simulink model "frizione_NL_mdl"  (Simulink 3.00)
settings: Solver=ode23s  StartTime=0.0  StopTime=10.0  RelTol=1e-10
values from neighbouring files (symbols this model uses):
  A = 4*(cm^2)    (= 0.0004)    [frizione_NL.m]
  b = 0.25*10^2*N*sec/m    (= 25)    [frizione_NL.m]
  Cm = 1*(cm^3)/(50*bar)    (= 2e-13)    [frizione_NL.m]
  Ic = Ic_max    (= 0.01)    [frizione_NL.m]
  K_x = [0:0.01:1]*3*mm    [frizione_NL.m]
  K_y = polyval(P,K_x)    [frizione_NL.m]
  mp = 0.3*Kg    (= 0.3)    [frizione_NL.m]
  P10 = 0*bar    (= 0)    [frizione_NL.m]
  Pm = 50*bar    (= 5000000)    [frizione_NL.m]
  x0 = 0*cm    (= 0)    [frizione_NL.m]

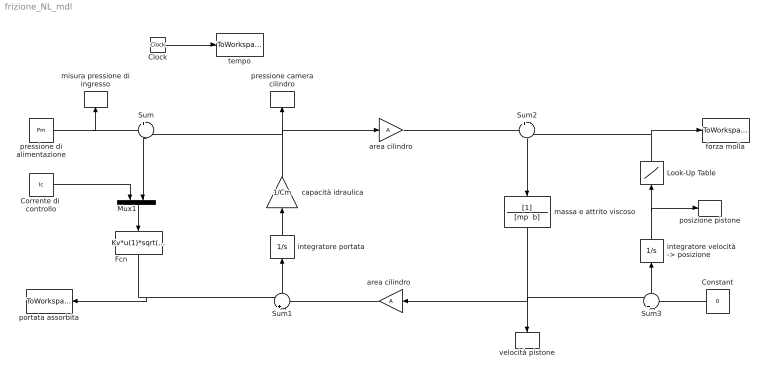
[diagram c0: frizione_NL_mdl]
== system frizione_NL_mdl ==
  Clock : Clock
  Constant : Constant  Orientation=left  Value=0
  Corrente di  controllo : Constant  Value=Ic
  Fcn : Fcn  Orientation=down  Expr=Kv*u(1)*sqrt(abs(u(2)))*((u(2)>=0)-(u(2)<0))
  Look-Up Table : Lookup  Orientation=up  InputValues=K_x  OutputValues=K_y
  Mux1 : Mux  Orientation=down  Inputs=2
  Sum : Sum  Orientation=down  Inputs=+-  SaturateOnIntegerOverflow=on
  Sum1 : Sum  Orientation=up  Inputs=+-  SaturateOnIntegerOverflow=on
  Sum2 : Sum  Orientation=down  Inputs=+-  SaturateOnIntegerOverflow=on
  Sum3 : Sum  Orientation=up  Inputs=+-  SaturateOnIntegerOverflow=on
  area cilindro : Gain  Gain=A  SaturateOnIntegerOverflow=on
  "area cilindro  " : Gain  Orientation=left  Gain=A  SaturateOnIntegerOverflow=on
  capacità idraulica : Gain  Orientation=up  Gain=1/Cm  SaturateOnIntegerOverflow=on
  forza molla : ToWorkspace  VariableName=Fm  SampleTime=-1  SaveFormat=Matrix
  integratore portata : Integrator  Orientation=up  ExternalReset=none  InitialConditionSource=internal  InitialCondition=P10  LimitOutput=off  UpperSaturationLimit=inf  LowerSaturationLimit=-inf  ShowSaturationPort=off  ShowStatePort=off  AbsoluteTolerance=auto
  "integratore velocità -> posizione" : Integrator  Orientation=up  ExternalReset=none  InitialConditionSource=internal  InitialCondition=x0  LimitOutput=off  UpperSaturationLimit=inf  LowerSaturationLimit=-inf  ShowSaturationPort=off  ShowStatePort=off  AbsoluteTolerance=auto
  massa e attrito viscoso : TransferFcn  Orientation=down  Numerator=[1]  Denominator="[mp  b]"
  misura pressione di ingresso : ToWorkspace  VariableName=P  SampleTime=-1  SaveFormat=Matrix
  portata assorbita : ToWorkspace  VariableName=Q  SampleTime=-1  SaveFormat=Matrix
  posizione pistone : ToWorkspace  VariableName=x  SampleTime=-1  SaveFormat=Matrix
  pressione camera cilindro : ToWorkspace  VariableName=P1  SampleTime=-1  SaveFormat=Matrix
  pressione di alimentazione : Constant  Value=Pm
  tempo : ToWorkspace  VariableName=t  SampleTime=-1  SaveFormat=Matrix
  velocità pistone : ToWorkspace  VariableName=xdot  SampleTime=-1  SaveFormat=Matrix
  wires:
  Sum1/1 -> integratore portata/1
  Sum3/1 -> "integratore velocità -> posizione"/1
  Sum2/1 -> massa e attrito viscoso/1
  area cilindro/1 -> Sum2/1
  "area cilindro  "/1 -> Sum1/2
  massa e attrito viscoso/1 -> Sum3/1, "area cilindro  "/1, velocità pistone/1
  Constant/1 -> Sum3/2
  Fcn/1 -> Sum1/1, portata assorbita/1
  capacità idraulica/1 -> area cilindro/1, Sum/2, pressione camera cilindro/1
  integratore portata/1 -> capacità idraulica/1
  Clock/1 -> tempo/1
  pressione di alimentazione/1 -> misura pressione di ingresso/1, Sum/1
  Sum/1 -> Mux1/2
  "integratore velocità -> posizione"/1 -> posizione pistone/1, Look-Up Table/1
  Look-Up Table/1 -> forza molla/1, Sum2/2
  Mux1/1 -> Fcn/1
  Corrente di  controllo/1 -> Mux1/1
